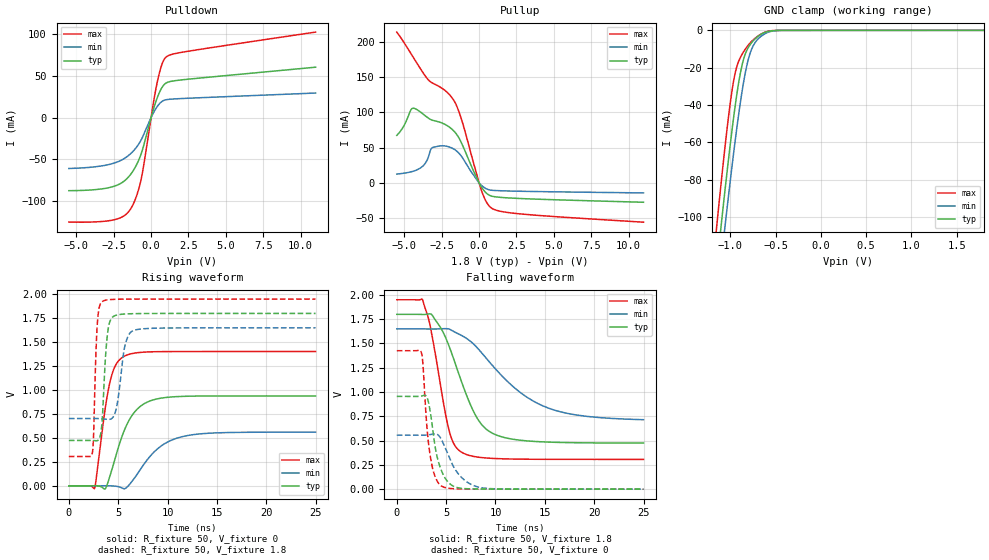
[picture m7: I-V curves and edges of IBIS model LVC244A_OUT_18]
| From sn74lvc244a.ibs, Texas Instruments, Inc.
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[Model]   LVC244A_OUT_18
Model_type  3-state
Enable   Active-Low
Vref =   0
Rref =   1000
Cref =   30p
Vmeas =   0.9
| variable   typ   min   max
C_comp   4.00pF   3.63pF   4.39pF
| C_pullup   7.31pF   4.25pF   10.61pF
| C_pulldown   7.92pF   3.85pF   14.08pF
| C_tri-state   4.00pF   3.63pF   4.39pF
[Temperature Range]   40   100   -40
| Ambient temperature   25   85   -40
[Voltage range]   1.8   1.65   1.95
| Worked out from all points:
|   slope of the pulldown table from 0 to 0.27 V, typ, clamps not added: 16.5 ohm
|   slope of the pullup table from 0 to 0.27 V, typ, clamps not added: 28.4 ohm
|   GND clamp passes 1 mA (typ) near -0.61 V on its own axis
|   rising waveform, R_fixture 50, V_fixture 0: 20-80 % time 2.1ns typ, 2.98ns min, 1.23ns max; typ from 0 V to 0.939 V
|   falling waveform, R_fixture 50, V_fixture 1.8: 20-80 % time 3.05ns typ, 5.84ns min, 1.73ns max; typ from 1.8 V to 0.474 V
|   rising waveform, R_fixture 50, V_fixture 1.8: 20-80 % time 453ps typ, 718ps min, 305ps max; typ from 0.474 V to 1.8 V
|   falling waveform, R_fixture 50, V_fixture 0: 20-80 % time 1.09ns typ, 1.84ns min, 747ps max; typ from 0.955 V to 0 V
[GND Clamp]
| LVC244A_OUT_18
|   Voltage   I(typ)   I(min)   I(max)
-5.5V     -2.404A    -2.35A     -2.478A
-1.15V    -126.2mA   -144.8mA   -104.1mA
-1.11V    -107.9mA   -126.9mA   -85.11mA
-1.07V    -90mA      -109.4mA   -66.84mA
-1.055V   -83.45mA   -102.9mA   -60.26mA
-965mV    -46.77mA   -65.85mA   -27.11mA
-875mV    -19.37mA   -33.78mA   -13.14mA
-820mV    -10.82mA   -19.09mA   -9.019mA
-775mV    -7.186mA   -11.23mA   -6.379mA
-655mV    -1.928mA   -2.966mA   -1.821mA
-430mV    -20.2uA    -30.69uA   -5.286uA
1.8V      55.22pA    18.39nA    22.67pA
[Pulldown]
| LVC244A_OUT_18
|   Voltage   I(typ)   I(min)   I(max)
-5.5V     -87.22mA   -60.73mA   -124.7mA
-2.615V   -82.71mA   -55.06mA   -122.5mA
-1.825V   -76.07mA   -49.17mA   -117.4mA
-1.325V   -66.69mA   -42.32mA   -107.6mA
-965mV    -56.01mA   -35.1mA    -93.01mA
-650mV    -42.45mA   -26.15mA   -72.29mA
170mV     10.71mA    6.134mA    19.19mA
490mV     27.22mA    15.13mA    48.55mA
765mV     36.88mA    19.69mA    65.36mA
1.035V    41.53mA    21.37mA    72.64mA
2.39V     45.62mA    23.01mA    78.89mA
11V       60.11mA    29.29mA    102mA
[Pullup]
| LVC244A_OUT_18
|   Voltage   I(typ)   I(min)   I(max)
-5.5V     67.37mA    12.28mA    214.3mA
-5.08V    78.92mA    13.34mA    201.5mA
-4.425V   105.9mA    16.22mA    179.4mA
-3.65V    96.16mA    26.1mA     153.6mA
-3.145V   89.1mA     49.54mA    142.2mA
-2.095V   80.77mA    51.55mA    127.9mA
-1.405V   65.91mA    43.3mA     104.5mA
140mV     -5.331mA   -3.219mA   -9.624mA
470mV     -14.4mA    -8.457mA   -26.5mA
805mV     -18.85mA   -10.63mA   -35.64mA
2.8V      -22.54mA   -12.19mA   -44.5mA
11V       -27.81mA   -14.55mA   -56.18mA
[Ramp]
| LVC244A_OUT_18
| variable   typ   min   max
dV/dt_r   0.58/2.13E-09   0.35/3.05E-09   0.86/1.25E-09
dV/dt_f   0.80/3.06E-09   0.56/5.84E-09   0.99/1.74E-09
R_load = 50
[Rising Waveform]
| LVC244A_OUT_18
R_fixture =   50
C_fixture =   0
L_fixture =   0
V_fixture =   0
V_fixture_min = 0
V_fixture_max = 0
|   Time   V(typ)   V(min)   V(max)
0s        303.2pV    3.871nV    100.1pV
2.605ns   848.2uV    18.27uV    -25.84mV
3.65ns    -34.64mV   737.6uV    784mV
4.135ns   94.52mV    299.7uV    1.071V
4.735ns   303.2mV    -3.525mV   1.259V
5.6ns     574.8mV    -30.4mV    1.352V
7.54ns    851.7mV    215.9mV    1.395V
9.17ns    912.6mV    402.2mV    1.401V
11.11ns   932.4mV    503mV      1.402V
24.99ns   938.9mV    560.6mV    1.402V
[Falling Waveform]
| LVC244A_OUT_18
R_fixture =   50
C_fixture =   0
L_fixture =   0
V_fixture =   1.8
V_fixture_min = 1.65
V_fixture_max = 1.95
|   Time   V(typ)   V(min)   V(max)
0s        1.8V       1.65V      1.95V
2.615ns   1.799V     1.65V      1.949V
3.39ns    1.805V     1.649V     1.677V
5.28ns    1.477V     1.649V     612.6mV
6.52ns    1.118V     1.585V     383.3mV
8.33ns    701.9mV    1.435V     328.5mV
10.32ns   548.6mV    1.202V     314.1mV
12.99ns   499mV      960.6mV    308.6mV
15.77ns   483.3mV    820.4mV    307.2mV
24.99ns   474.4mV    715.2mV    306.6mV
[Rising Waveform]
| LVC244A_OUT_18
R_fixture =   50
C_fixture =   0
L_fixture =   0
V_fixture =   1.8
V_fixture_min = 1.65
V_fixture_max = 1.95
|   Time   V(typ)   V(min)   V(max)
0s        473.9mV    702.8mV    306.6mV
2.39ns    473.5mV    703mV      348.6mV
2.505ns   472.8mV    703.1mV    531.4mV
2.88ns    472.1mV    702.7mV    1.687V
3.425ns   769.8mV    698.9mV    1.927V
3.92ns    1.591V     694.4mV    1.942V
4.605ns   1.774V     740mV      1.947V
5.675ns   1.794V     1.46V      1.949V
6.535ns   1.797V     1.622V     1.95V
24.99ns   1.8V       1.65V      1.95V
[Falling Waveform]
| LVC244A_OUT_18
R_fixture =   50
C_fixture =   0
L_fixture =   0
V_fixture =   0
V_fixture_min = 0
V_fixture_max = 0
|   Time   V(typ)   V(min)   V(max)
0s        955.1mV    555.8mV    1.425V
2.495ns   958mV      555.4mV    1.405V
2.66ns    962.9mV    555.3mV    1.272V
3.065ns   944.5mV    557.2mV    626.5mV
3.37ns    809.6mV    561.8mV    356.5mV
3.98ns    384.5mV    568.6mV    107mV
4.565ns   181.4mV    502.2mV    30.08mV
6.185ns   14.79mV    164.1mV    2.825mV
8.305ns   1.927mV    20.19mV    635.3uV
24.99ns   59.85uV    164.4uV    24.01uV
